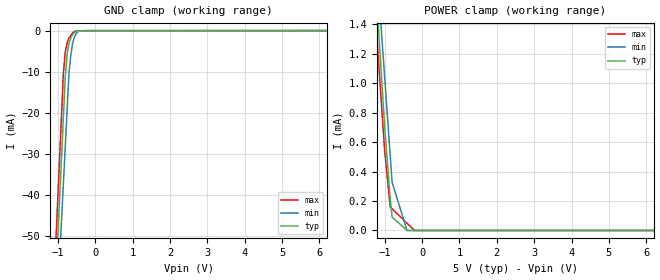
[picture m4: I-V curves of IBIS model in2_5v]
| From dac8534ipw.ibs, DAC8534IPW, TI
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[Model] in2_5v
Model_type Input
Vinl = 800.000mV
Vinh = 2.40000V
C_comp 2.00000pF 2.00000pF 2.00000pF
| variable typ   min   max
[Voltage Range] 5.00000V 4.50000V 5.50000V
[POWER Clamp Reference] 5.00000V 4.50000V 5.50000V
[GND Clamp Reference] 0.00000V 0.00000V 0.00000V
[Temperature Range]   25   105   -40
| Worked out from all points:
|   GND clamp passes 1 mA (typ) near -0.61 V on its own axis
[GND Clamp]
-5V       -833.8mA   -786.1mA   -855.4mA
-850mV    -21.2mA    -37.48mA   -10.47mA
-800mV    -11.41mA   -28.46mA   -5.251mA
-750mV    -5.806mA   -19.44mA   -2.945mA
-700mV    -2.959mA   -10.42mA   -1.792mA
-650mV    -1.695mA   -5.998mA   -1.149mA
-600mV    -888.5uA   -2.974mA   -505.5uA
-550mV    -392uA     -1.411mA   -163.1uA
-500mV    -126.7uA   -629.5uA   -33.48uA
-450mV    -27.92uA   -237.9uA   -26.94uA
-200mV    -1.028uA   -1.23uA    -659.6nA
10V       9.897uA    20.27uA    21.95uA
[POWER Clamp]
-5V       16.91mA    15.39mA    15.4mA
-1.4V     2.326mA    2.479mA    2.028mA
-1V       706uA      1.045mA    543.1uA
-850mV    212.3uA    506.6uA    159.5uA
-800mV    91.19uA    327.2uA    147.2uA
-700mV    68.39uA    245.4uA    122.7uA
-400mV    0A         0A         49.06uA
-300mV    0A         0A         24.53uA
-200mV    0A         0A         0A
-100mV    0A         0A         0A
10V       0A         0A         0A
